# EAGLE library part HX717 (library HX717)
SOP-16 Analog To Digital Converters (ADCs) ROHS Source: Datasheet
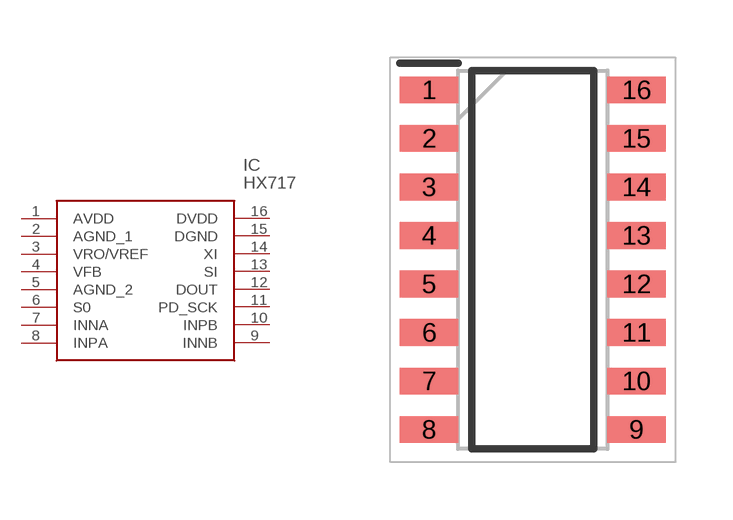
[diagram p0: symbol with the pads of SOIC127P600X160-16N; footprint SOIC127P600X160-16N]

Designator prefix IC

## HX717 (Description: SOP-16 Analog To Digital Converters (ADCs) ROHS; Height: 1.6mm; Manufacturer_Name: AVIA; Manufacturer_Part_Number: HX717)  [SOIC127P600X160-16N]
1  AVDD
2  AGND_1
3  VRO/VREF
4  VFB
5  AGND_2
6  S0
7  INNA
8  INPA
9  INNB
10  INPB
11  PD_SCK
12  DOUT
13  SI
14  XI
15  DGND
16  DVDD

## Footprint SOIC127P600X160-16N (pad centres in mm)
HX717
smd 1.525 x 0.7: 1 -2.712,4.445; 2 -2.712,3.175; 3 -2.712,1.905; 4 -2.712,0.635; 5 -2.712,-0.635; 6 -2.712,-1.905; 7 -2.712,-3.175; 8 -2.712,-4.445; 9 2.712,-4.445; 10 2.712,-3.175; 11 2.712,-1.905; 12 2.712,-0.635; 13 2.712,0.635; 14 2.712,1.905; 15 2.712,3.175; 16 2.712,4.445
